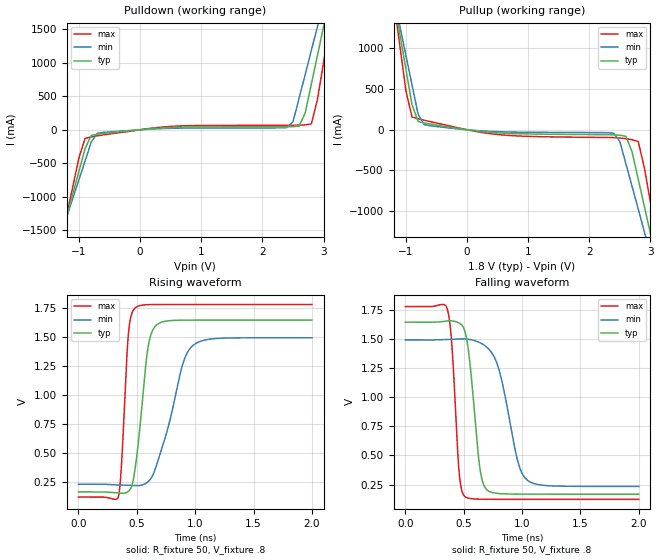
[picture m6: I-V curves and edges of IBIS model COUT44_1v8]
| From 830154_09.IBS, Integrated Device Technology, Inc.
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| 2.45455e+00   -4.20356e-03   -5.32096e-01   -1.21525e-04
| 2.50909e+00   -7.71540e-03   -1.06712e+00   -4.40197e-04
| 2.56364e+00   -1.61062e-02   -1.60245e+00   -1.36751e-03
| 2.61818e+00   -5.97340e-02   -2.13803e+00   -3.36870e-03
| 2.67273e+00   -3.85760e-01   -2.67384e+00   -6.58445e-03
| 2.72727e+00   -1.02850e+00   -3.20984e+00   -1.08472e-02
| 2.78182e+00   -1.67153e+00   -3.74599e+00   -1.64545e-02
| 2.83636e+00   -2.31480e+00   -4.28227e+00   -3.18148e-02
| 2.89091e+00   -2.95826e+00   -4.81866e+00   -1.86961e-01
| 2.94545e+00   -3.60187e+00   -5.35516e+00   -9.59692e-01
| 3.00000e+00   -4.24560e+00   -5.89173e+00   -1.78158e+00
| 3.05455e+00   -4.88944e+00   -6.42838e+00   -2.60363e+00
| 3.10909e+00   -5.53337e+00   -6.96509e+00   -3.42581e+00
| 3.16364e+00   -6.17736e+00   -7.50186e+00   -4.24809e+00
| 3.21818e+00   -6.82142e+00   -8.03867e+00   -5.07044e+00
| 3.27273e+00   -7.46552e+00   -8.57552e+00   -5.89285e+00
| 3.32727e+00   -8.10966e+00   -9.11241e+00   -6.71531e+00
| 3.38182e+00   -8.75383e+00   -9.64932e+00   -7.53780e+00
| 3.43636e+00   -9.39803e+00   -1.01863e+01   -8.36031e+00
| 3.49091e+00   -1.00423e+01   -1.07232e+01   -9.18283e+00
| 3.54545e+00   -1.06865e+01   -1.12602e+01   -1.00054e+01
| 3.60000e+00   -1.13307e+01   -1.17972e+01   -1.08279e+01
[Model] COUT44_1v8
Model_type   Output
Polarity   Non-Inverting
Vmeas = 1.1
Rref = 50
Cref = 0
Vref = .9
|   typ   min   max
C_comp   2pF   1.5pF   2.5pF
|   typ   min   max
[Voltage range]  1.8V   1.710V   1.890V
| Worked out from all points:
|   slope of the pulldown table from 0 to 0.27 V, typ, clamps not added: 12.4 ohm
|   slope of the pullup table from 0 to 0.27 V, typ, clamps not added: 11.3 ohm
|   rising waveform, R_fixture 50, V_fixture .8: 20-80 % time 89.2ps typ, 190ps min, 49.8ps max; typ from 0.167 V to 1.64 V
|   falling waveform, R_fixture 50, V_fixture .8: 20-80 % time 82.4ps typ, 154ps min, 54.6ps max; typ from 1.64 V to 0.167 V
[pulldown]
|Voltage   I (typ)   I (min)   I (max)
-3.3V     -8.339A    -7.182A    -10.24A
-1.3V     -1.626A    -1.582A    -1.703A
-900mV    -280.8mA   -464.6mA   -130.1mA
-700mV    -66.79mA   -52.64mA   -91.41mA
2.4V      45.81mA    32.11mA    67.39mA
2.5V      46.94mA    119.3mA    67.77mA
2.7V      252.9mA    828.7mA    73.03mA
2.8V      682mA      1.186A     87.73mA
2.9V      1.112A     1.544A     453.7mA
3V        1.544A     1.902A     1.005A
3.1V      1.976A     2.261A     1.558A
6.6V      17.45A     15.1A      21.32A
[pullup]
|Voltage   I (typ)   I (min)   I (max)
-3.3V     10.82A     9.291A     13.32A
-1.2V     1.621A     1.64A      1.6A
-1.1V     1.183A     1.277A     1.04A
-900mV    308.9mA    551.5mA    156.6mA
-700mV    83.38mA    62.39mA    116.4mA
2.4V      -62.57mA   -42.43mA   -96.66mA
2.6V      -80.74mA   -420.9mA   -110.7mA
2.8V      -605.9mA   -973.1mA   -144.8mA
2.9V      -939.6mA   -1.25A     -465mA
3V        -1.274A    -1.528A    -892mA
3.1V      -1.609A    -1.806A    -1.319A
6.6V      -13.35A    -11.6A     -16.26A
[Ramp]
|   typ   min   max
dV/dt_r   1.19/.138n   1.01/.281n   1.34/.0774n
dV/dt_f   1.19/.128n   1.01/.249n   1.34/.085n
[Rising Waveform]
R_fixture = 50
V_fixture = .8
V_fixture_max = .945
V_fixture_min = .855
C_fixture = 0.0p
| Time   typ   min   max
0s        167.4mV    233.8mV    123.4mV
342.3ps   158.7mV    227.4mV    129.1mV
367.5ps   156.2mV    226.5mV    383.2mV
428.4ps   172.9mV    223.7mV    1.533V
489.3ps   396.5mV    221.4mV    1.752V
592.2ps   1.386V     250.9mV    1.776V
672ps     1.604V     407.3mV    1.778V
894.6ps   1.643V     1.27V      1.778V
982.8ps   1.644V     1.428V     1.778V
1.999ns   1.644V     1.492V     1.778V
[Falling Waveform]
R_fixture = 50
V_fixture = .8
V_fixture_max = .945
V_fixture_min = .855
C_fixture = 0.0p
| Time   typ   min   max
0s        1.644V     1.492V     1.778V
359.1ps   1.655V     1.495V     1.757V
399ps     1.655V     1.497V     1.441V
462ps     1.636V     1.501V     341.8mV
510.3ps   1.564V     1.5V       147mV
636.3ps   407.5mV    1.469V     124.6mV
697.2ps   205.8mV    1.43V      123.7mV
798ps     173.4mV    1.249V     123.4mV
1.039ns   167.7mV    292.3mV    123.4mV
1.999ns   167.4mV    233.9mV    123.4mV
